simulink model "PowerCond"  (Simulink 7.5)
settings: Solver=ode45  StartTime=0.0  StopTime=10.0  RelTol=1e-3

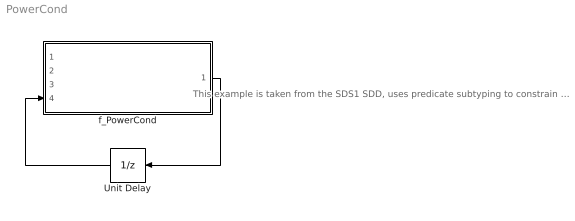
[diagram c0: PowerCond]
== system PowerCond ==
  note: This example is taken from the SDS1 SDD, uses predicate subtyping to constrain Kout > Kin. Table is 1 Dimensional Horizontal provable in both PVS and CVC3
  Unit Delay : UnitDelay  SampleTime=-1
  f_PowerCond : Subsystem
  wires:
  f_PowerCond/1(output) -> Unit Delay/1
  Unit Delay/1 -> f_PowerCond/4(Prev)

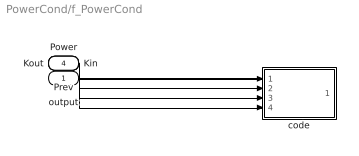
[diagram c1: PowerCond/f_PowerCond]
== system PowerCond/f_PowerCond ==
  Power : Inport  OutDataType=fixdt(1, 16)  OutScaling=2^0
  Kin : Inport  Port=2  OutDataType=fixdt(1, 16)  OutScaling=2^0
  Kout : Inport  Port=3  OutDataType=fixdt(1, 16)  OutScaling=2^0
  Prev : Inport  Port=4  OutDataType=fixdt(1, 16)  OutScaling=2^0
  code : Stateflow chart  TreatAsAtomicUnit=on
  output : Outport  OutDataType=fixdt(1, 16)  OutScaling=2^0
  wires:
  Power/1 -> code/1(Power)
  Kin/1 -> code/2(Kin)
  Kout/1 -> code/3(Kout)
  Prev/1 -> code/4(Prev)
  code/1(output) -> output/1

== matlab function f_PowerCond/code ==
function output  = f_PowerCond(Power,Kin,Kout,Prev)
%%#eml
output=false;
if(Power<Kout)
  output = false;
elseif(Kout<=Power && Power<=Kin)
  output = Prev;
elseif(Kin<Power)
  output = true;
end
